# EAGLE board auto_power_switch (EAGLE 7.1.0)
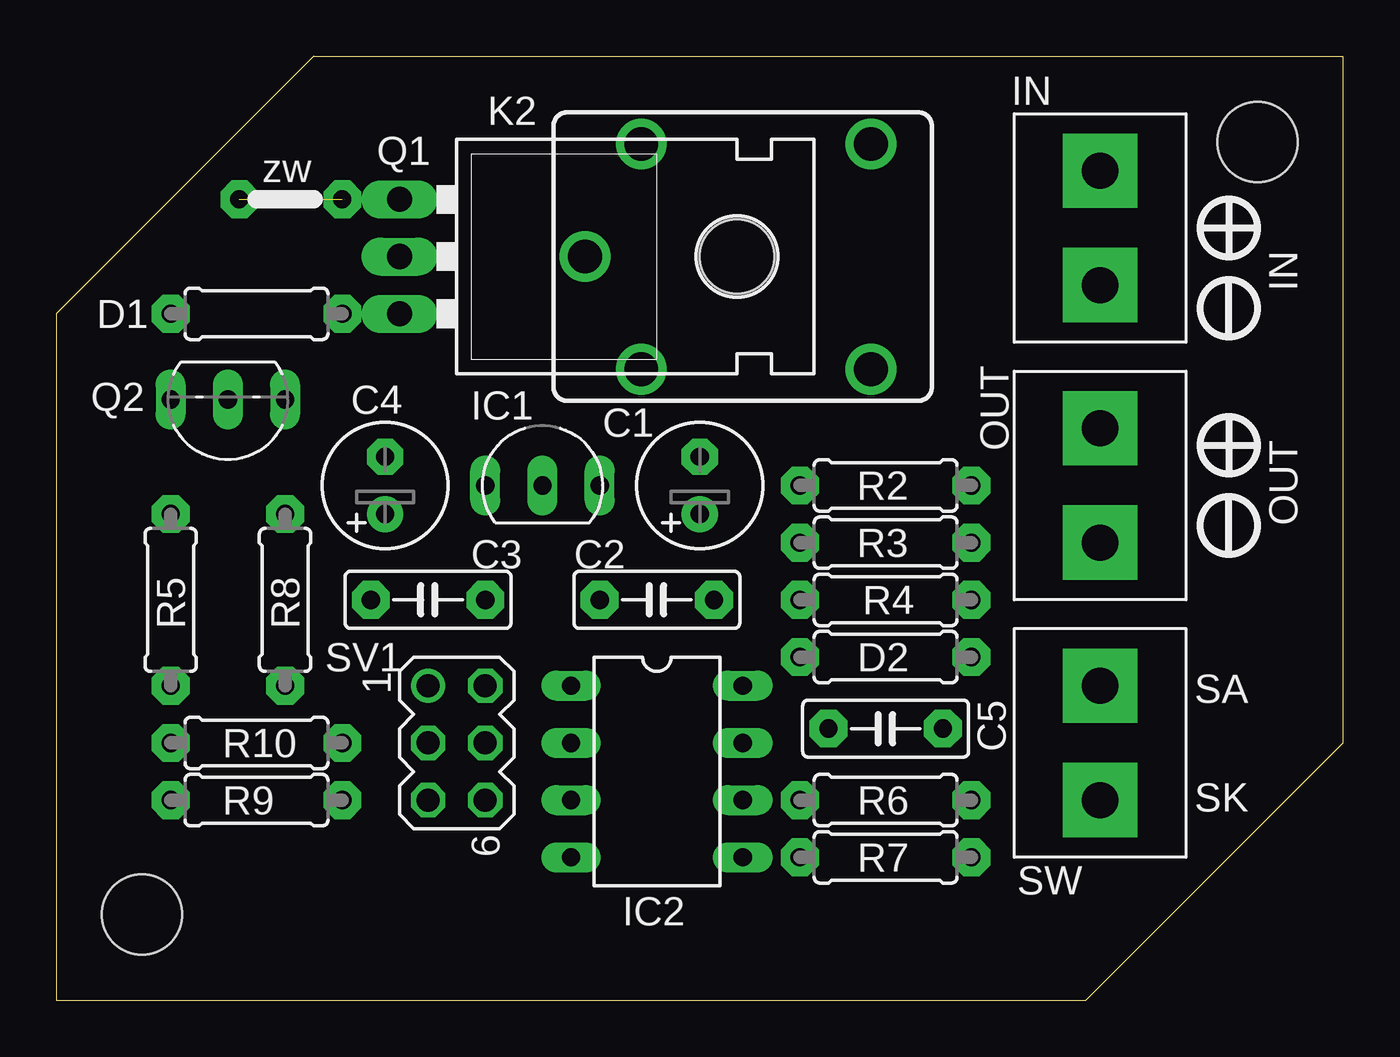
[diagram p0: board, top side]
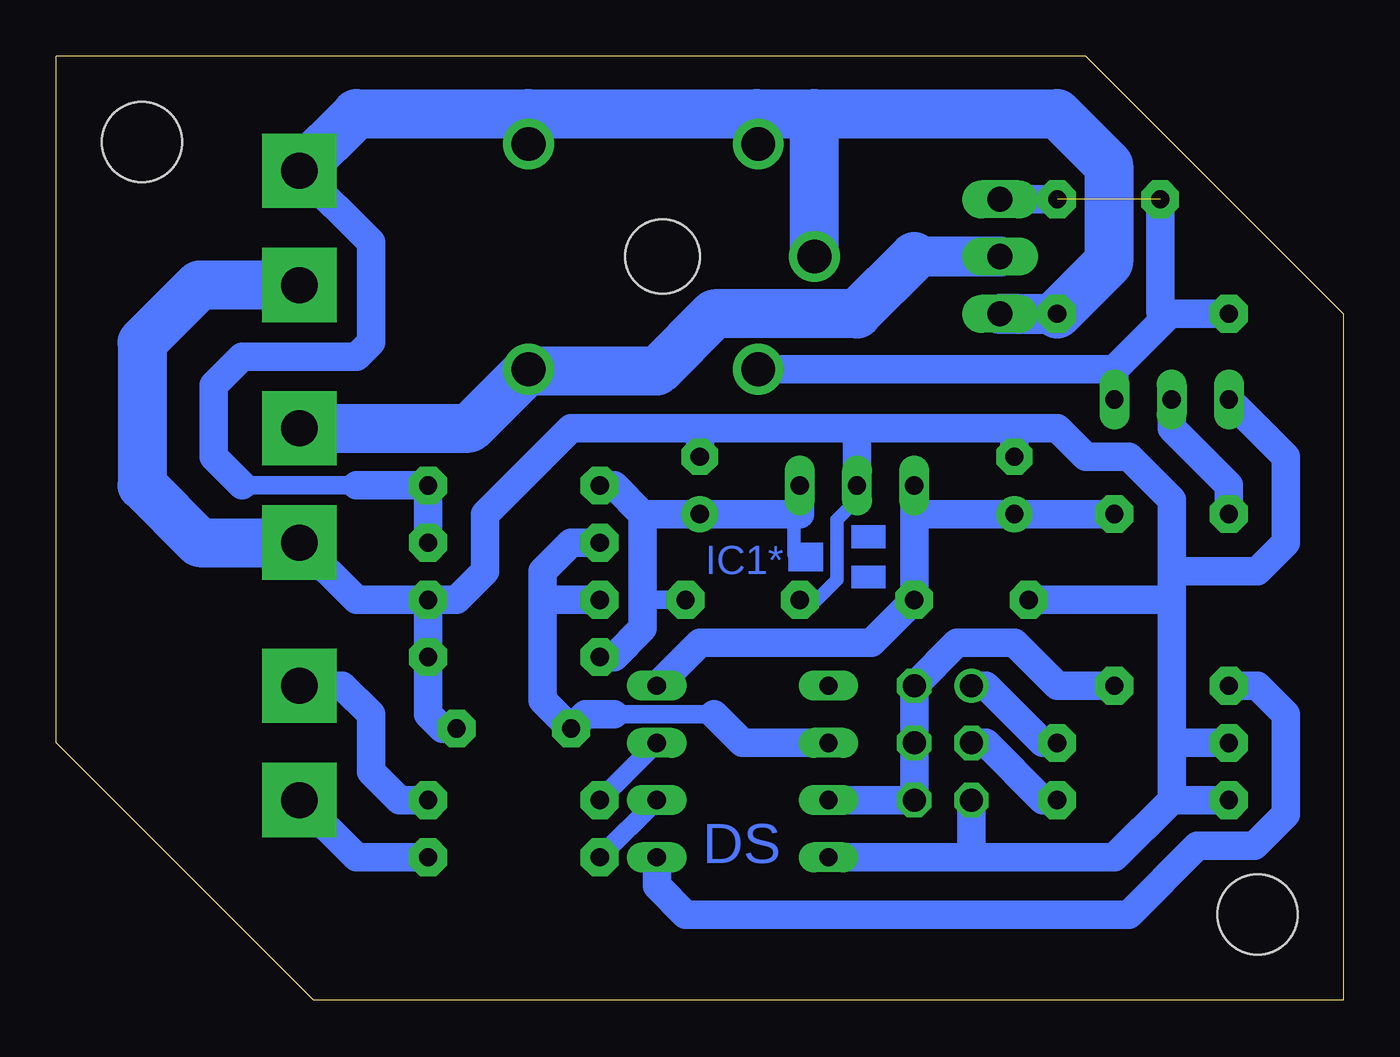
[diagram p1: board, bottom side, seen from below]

Size 57.15 x 41.91 mm. Coordinates in mm from the lower left corner, seen from the top.
Outline: 0,0 45.72,0 57.15,11.43 57.15,41.91 11.43,41.91 0,30.48 0,0
Copper layers (1*16): Top 0.035mm / dielectric 1.5mm / Bottom 0.035mm
Design rules "default": minimum track width 10mil, minimum drill 24mil, track to track 8mil, track to pad 8mil, pad to pad 8mil, via to via 8mil, smd to smd 8mil, copper to edge 40mil, drill to drill 8mil, minimum pad ring 10mil, minimum via ring 8mil, stop-mask expansion 4mil, vias tented up to drill 0mil, thermal gap 10mil
Holes 3.56 mm at 3.81,3.81 53.34,38.1

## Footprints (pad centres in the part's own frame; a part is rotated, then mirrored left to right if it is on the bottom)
E2,5-6 = drill 0.813 pad 1.6: + -1.27,0 | drill 0.813 pad 1.6 octagon: - 1.27,0
C050-025X075 = drill 0.813 pad 1.676 octagon: 1 -2.54,0; 2 2.54,0
0207/7 = drill 0.813 pad 1.676 octagon: 1 -3.81,0; 2 3.81,0
TO92 = drill 0.813 pad 1.27 long: 1 -2.54,0; 2 0,0; 3 2.54,0
DIL08 = drill 0.813 long: 1 -3.81,-3.81; 2 -1.27,-3.81; 3 1.27,-3.81; 4 3.81,-3.81; 5 3.81,3.81; 6 1.27,3.81; 7 -1.27,3.81; 8 -3.81,3.81
ARK2/500 = drill 1.6 pad 3.302 square: 1 -2.54,0; 2 2.54,0
CQ1 = drill 1.5: 1 4.5,-5; 2 4.5,5; C 7,0; NC -5.7,-5; NO -5.7,5
TO220BHS = drill 1.118 long: D 0,-3.81; G -2.54,-3.81; S 2.54,-3.81 | hole 3.302: 0,11.176
TO92-EBC = drill 0.813 long: B 0,-1.27; C -2.54,-1.27; E 2.54,-1.27
MA03-2 = drill 1.016: 1 -2.54,-1.27 | drill 1.016 octagon: 2 -2.54,1.27; 3 0,-1.27; 4 0,1.27; 5 2.54,-1.27; 6 2.54,1.27

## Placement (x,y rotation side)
C1  100uF  [E2,5-6]  28.57,22.86 90 top
C2  100nF  [C050-025X075]  26.67,17.78 180 top
C3  100nF  [C050-025X075]  16.51,17.78 180 top
C4  100uF  [E2,5-6]  14.61,22.86 90 top
C5  100nF  [C050-025X075]  36.83,12.06 180 top
D1  1N5819  [0207/7]  8.89,30.48 0 top
D2  24V  [0207/7]  36.83,15.24 0 top
IC1  LP2931ACZ-5.0  [TO92]  21.59,22.86 0 top
IC2  ATTINY45  [DIL08]  26.67,10.16 270 top
IN  ARK2ARK2/500  [ARK2/500]  46.35,34.29 90 top
K2  CQ1-12V  [CQ1]  30.48,33.02 180 top
OUT  ARK2ARK2/500  [ARK2/500]  46.35,22.86 270 top
Q1  [TO220BHS]  19.05,33.02 270 top
Q2  BC546B  [TO92-EBC]  7.62,25.4 180 top
R2  10R  [0207/7]  36.83,22.86 180 top
R3  909k  [0207/7]  36.83,20.32 180 top
R4  100k  [0207/7]  36.83,17.78 180 top
R5  5.1k  [0207/7]  5.08,17.78 270 top
R6  220R  [0207/7]  36.83,8.89 0 top
R7  220R  [0207/7]  36.83,6.35 0 top
R8  100k  [0207/7]  10.16,17.78 270 top
R9  10k  [0207/7]  8.89,8.89 0 top
R10  5.1k  [0207/7]  8.89,11.43 0 top
SV1  [MA03-2]  17.78,11.43 270 top
SW  ARK2ARK2/500  [ARK2/500]  46.35,11.43 270 top

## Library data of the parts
C1-C5 D1 D2 R2-R10 = rcl
IC1 = v-reg
IC2 = avr-7
IN OUT SW = dimmer
K2 = relay; OC_FARNELL: unknown; OC_NEWARK: unknown
Q1 = transistor-power
Q2 = transistor-npn
SV1 = con-lstb; OC_FARNELL: unknown; OC_NEWARK: unknown

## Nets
GND: C1.- C2.2 C3.2 C4.- C5.1 D2.2 IC1.2 IC2.4 IN.1 OUT.2 Q2.E R4.1 R9.1 R10.1 SV1.5
N$1: R10.2 SV1.1
N$2: R9.2 SV1.3
N$5: Q2.B R5.1
N$7: R6.2 SW.1
N$8: R7.2 SW.2
N$9: D1.1 K2.2 Q1.G Q2.C
OUT: IC2.5 R5.2
SA: IC2.7 R6.1
SK: IC2.6 R7.1
VAN: C5.2 IC2.2 R3.2 R4.2
VCF: IC2.3 R8.2 SV1.2 SV1.4 SV1.6
VDD: C3.1 C4.+ IC1.1 IC2.8 R8.1
VM: D1.2 IN.2 K2.1 K2.C K2.NC Q1.S R2.1 R3.1
VO: K2.NO OUT.1 Q1.D
VST: C1.+ C2.1 D2.1 IC1.3 R2.2

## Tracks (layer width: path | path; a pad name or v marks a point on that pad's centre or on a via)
GND
  Bottom 0.61: 22.48,18.67 22.48,21.34 21.59,22.23 IC1.2 | 22.5,18.69 22.48,18.67 | 22.48,18.67 23.37,17.78 C2.2
  Bottom 1.27: IC2.4 16.51,6.35 | SV1.5 16.51,6.35 | 7.62,8.89 10.16,6.35 16.51,6.35 | R4.1 D2.2 40.64,12.7 40,12.06 C5.1 | R4.1 43.81,17.78 OUT.2 | R4.1 39.37,17.78 38.1,19.05 38.1,21.59 34.29,25.4 28.57,25.4 | 28.57,25.4 21.59,25.4 | 21.59,25.4 14.61,25.4 | 14.61,25.4 12.7,25.4 11.43,24.13 9.53,24.13 7.62,22.23 7.62,19.05 | C1.- 28.57,25.4 | IC1.2 21.59,25.4 | Q2.E 2.54,24.13 2.54,20.32 3.81,19.05 7.62,19.05 | C4.- 14.61,25.4 | 7.62,8.89 7.62,11.43 | 7.62,11.43 7.62,17.78 | 7.62,17.78 7.62,19.05 | R9.1 7.62,8.89 | R10.1 7.62,11.43 | C3.2 7.62,17.78
  Bottom 2.184: IN.1 50.8,31.75 53.34,29.21 53.34,22.86 50.8,20.32 OUT.2
N$1
  Bottom 1.27: SV1.1 15.87,13.97 13.33,11.43 R10.2
N$2
  Bottom 1.27: SV1.3 15.87,11.43 13.33,8.89 R9.2
N$5
  Bottom 1.27: Q2.B 7.62,25.4 5.08,22.86 R5.1
N$7
  Bottom 1.27: R6.2 41.91,8.89 43.18,10.16 43.18,12.7 44.45,13.97 SW.1
N$8
  Bottom 1.27: R7.2 43.81,6.35 SW.2
N$9  (via drill 0.8 pad 1.68)  (1 unrouted)
  Bottom 1.27: K2.2 10.16,28.02 | Q2.C 10.16,28.02 | D1.1 7.7,30.48 | 7.7,30.48 10.16,28.02 | Q1.G v12.7,35.56 | v8.13,35.56 8.13,30.56 7.7,30.48
OUT
  Bottom 1.27: IC2.5 30.48,5.08 29.21,3.81 9.53,3.81 6.48,6.86 3.94,6.86 2.54,8.26 2.54,12.7 3.81,13.97 R5.2
SA
  Bottom 0.813: IC2.7 R6.1
SK
  Bottom 0.813: IC2.6 R7.1
VAN
  Bottom 0.813: 27.94,12.7 32.39,12.7
  Bottom 1.27: R3.2 34.29,20.32 35.56,19.05 35.56,17.78 | 35.56,17.78 35.56,13.34 C5.2 33.66,12.7 32.39,12.7 | R4.2 35.56,17.78 | IC2.2 26.67,11.43 27.94,12.7
VCF
  Bottom 1.27: IC2.3 SV1.6 SV1.4 SV1.2 17.14,15.88 14.61,15.88 12.7,13.97 R8.2
VDD
  Bottom 0.61: 19.16,20.69 19.05,20.57
  Bottom 1.27: R8.1 C4.+ 19.05,21.59 | IC2.8 28.57,15.88 20.96,15.88 C3.1 19.05,20.57 19.05,21.59 | 19.05,21.59 IC1.1
VM
  Bottom 0.813: 48.89,22.86 43.81,22.86
  Bottom 1.27: 48.89,22.86 50.16,24.13 50.16,27.3 48.89,28.58 43.81,28.58 43.18,29.21 43.18,33.65 IN.2 | 43.81,22.86 R2.1 R3.1
  Bottom 1.778: Q1.S D1.2
  Bottom 2.184: 26.04,39.37 23.5,39.37 | 23.5,39.37 12.7,39.37 10.41,37.08 10.41,32.77 D1.2 | K2.1 25.98,39.32 26.04,39.37 | K2.C 23.48,39.35 23.5,39.37 | IN.2 43.81,39.37 36.19,39.37 | 36.19,39.37 26.04,39.37 | K2.NC 36.18,39.35 36.19,39.37
VO
  Bottom 1.778: Q1.D 19.05,33.02
  Bottom 2.184: 19.05,33.02 21.59,30.48 27.94,30.48 30.48,27.94 36.1,27.94 K2.NO 38.8,25.4 OUT.1
VST
  Bottom 0.61: 24.26,19.69 24.38,19.81 24.38,21.84 24.13,22.1
  Bottom 0.813: C2.1 31.11,17.78
  Bottom 1.27: R2.2 32.39,22.86 31.11,21.59 | 31.11,21.59 31.11,17.78 31.11,16.51 32.39,15.24 D2.1 | IC1.3 24.13,22.1 24.13,21.59 C1.+ 31.11,21.59
(copper drawn outside any net)
  shapes: Bottom area x3

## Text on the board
Bottom: IC1* | DS
tPlace: zw | IN | OUT | SA | SK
